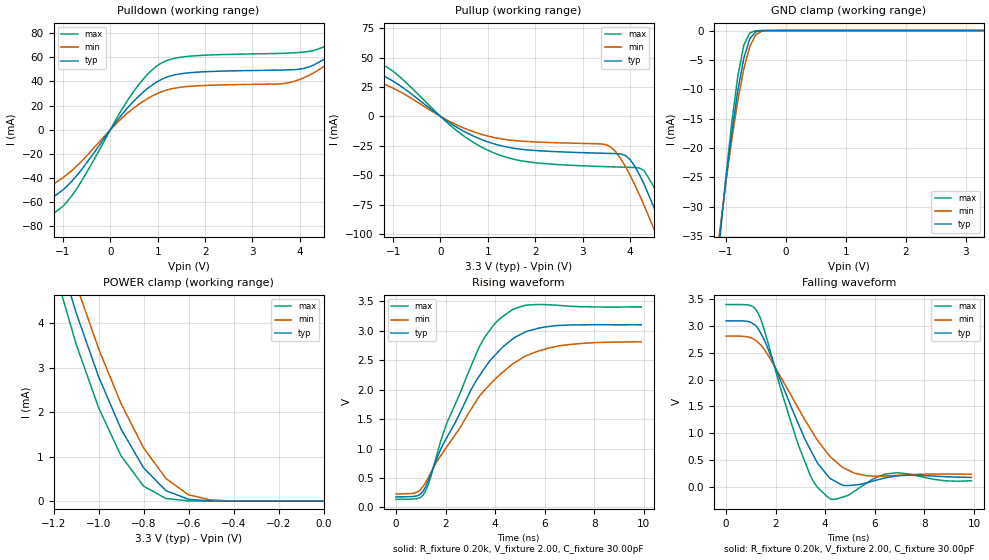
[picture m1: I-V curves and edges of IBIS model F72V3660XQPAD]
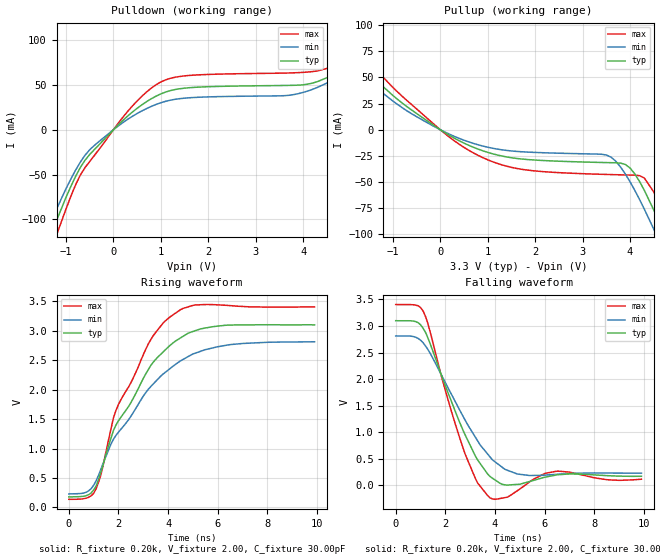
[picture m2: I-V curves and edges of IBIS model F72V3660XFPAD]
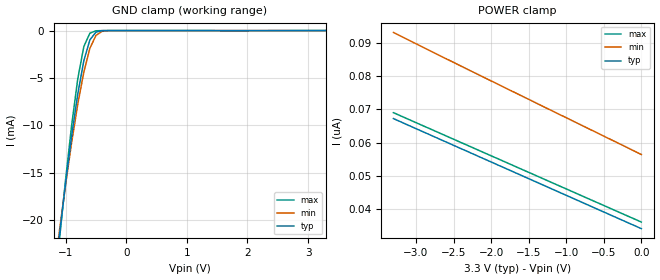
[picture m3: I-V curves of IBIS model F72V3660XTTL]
| IBIS file 72v3660p.ibs created by s2ibis2 version 1.1
| North Carolina State University Electronics Research Laboratory  1995
[IBIS ver]   2.1
[File name]   72v3660p.ibs
[File Rev]   1.0
[Date]   08/30/2001
[Source]   Integrated Device Technology, Inc.
[Notes]   1. Temperatures: typ=25C, min=85C, max=-40C 2. Cemos11.5_3v
   process. 3. Ramp rates based on 50 ohm load.
[Copyright]   Copyright 1999, Integrated Device Technology, Inc.
|   Component idt72v3660x
[Component]   idt72v3660x
[Manufacturer]   Integrated Device Technology
[Package]
| variable   typ   min   max
R_pkg   0.75   0.60   0.90
L_pkg   8.10nH   8.30nH   9.90nH
C_pkg   0.53pF   0.46pF   0.60pF
[Pin]  signal_name   model_name   R_pin   L_pin   C_pin
1   D0   F72V3660XTTL
2   D1   F72V3660XTTL
3   D2   F72V3660XTTL
4   D3   F72V3660XTTL
5   D4   F72V3660XTTL
6   D5   F72V3660XTTL
7   D6   F72V3660XTTL
8   D7   F72V3660XTTL
9   D8   F72V3660XTTL
10   D9   F72V3660XTTL
11   D10   F72V3660XTTL
12   D11   F72V3660XTTL
13   D12   F72V3660XTTL
14   D13   F72V3660XTTL
15   D14   F72V3660XTTL
16   D15   F72V3660XTTL
17   D16   F72V3660XTTL
18   D17   F72V3660XTTL
19   D18   F72V3660XTTL
20   D19   F72V3660XTTL
21   D20   F72V3660XTTL
22   D21   F72V3660XTTL
23   D22   F72V3660XTTL
24   D23   F72V3660XTTL
25   D24   F72V3660XTTL
26   D25   F72V3660XTTL
27   D26   F72V3660XTTL
28   D27   F72V3660XTTL
29   D28   F72V3660XTTL
30   D29   F72V3660XTTL
31   D30   F72V3660XTTL
32   D31   F72V3660XTTL
33   D32   F72V3660XTTL
34   D33   F72V3660XTTL
35   D34   F72V3660XTTL
36   D35   F72V3660XTTL
37   GND   GND
38   WENL   F72V3660XTTL
39   WCLK   F72V3660XTTL
40   PRSL   F72V3660XTTL
41   MRSL   F72V3660XTTL
42   LDL   F72V3660XTTL
43   FWFTSI   F72V3660XTTL
44   FFL   F72V3660XFPAD
45   PAFL   F72V3660XFPAD
46   OW   F72V3660XTTL
47   FSEL0   F72V3660XTTL
48   HFL   F72V3660XFPAD
49   FSEL1   F72V3660XTTL
50   BEL   F72V3660XTTL
51   IP   F72V3660XTTL
52   BM   F72V3660XTTL
53   ASYRL   F72V3660XTTL
54   VCC   POWER
55   PAEL   F72V3660XFPAD
56   PFM   F72V3660XTTL
57   EFL   F72V3660XFPAD
58   MARK   F72V3660XTTL
59   RCLK   F72V3660XTTL
60   RENL   F72V3660XTTL
61   RTL   F72V3660XTTL
62   OEL   F72V3660XTTL
63   Q0   F72V3660XQPAD
64   Q1   F72V3660XQPAD
65   Q2   F72V3660XQPAD
66   Q3   F72V3660XQPAD
67   Q4   F72V3660XQPAD
68   Q5   F72V3660XQPAD
69   Q6   F72V3660XQPAD
70   Q7   F72V3660XQPAD
71   Q8   F72V3660XQPAD
72   Q9   F72V3660XQPAD
73   Q10   F72V3660XQPAD
74   Q11   F72V3660XQPAD
75   Q12   F72V3660XQPAD
76   Q13   F72V3660XQPAD
77   Q14   F72V3660XQPAD
78   Q15   F72V3660XQPAD
79   Q16   F72V3660XQPAD
80   Q17   F72V3660XQPAD
81   Q18   F72V3660XQPAD
82   Q19   F72V3660XQPAD
83   Q20   F72V3660XQPAD
84   Q21   F72V3660XQPAD
85   Q22   F72V3660XQPAD
86   Q23   F72V3660XQPAD
87   Q24   F72V3660XQPAD
88   Q25   F72V3660XQPAD
89   Q26   F72V3660XQPAD
90   Q27   F72V3660XQPAD
91   Q28   F72V3660XQPAD
92   Q29   F72V3660XQPAD
93   Q30   F72V3660XQPAD
94   Q31   F72V3660XQPAD
95   Q32   F72V3660XQPAD
96   Q33   F72V3660XQPAD
97   Q34   F72V3660XQPAD
98   Q35   F72V3660XQPAD
99   TDO   F72V3660XQPAD
100   IW   F72V3660XTTL
101   SENL   F72V3660XTTL
102   ASYWL   F72V3660XTTL
| Models and submodels in the file (3): F72V3660XQPAD (3-state), F72V3660XFPAD (Output), F72V3660XTTL (Input)
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| FIN  FIN   dummy_model
| QIN  QIN   dummy_model
| QOEL QOEL   dummy_model
|   Model F72V3660XQPAD
[Model]   F72V3660XQPAD
Model_type   3-state
Polarity   Non-Inverting
Enable   Active-Low
Vinl =  0.000V
Vinh =  3.000V
Vmeas =  1.500V
C_comp   3.00pF   NA   NA
[Temperature Range]   25.00   85.00   -40.00
[Voltage Range]   3.30V   3.00V   3.60V
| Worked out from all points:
|   slope of the pulldown table from 0 to 0.495 V, typ, clamps not added: 20.9 ohm
|   slope of the pullup table from 0 to 0.495 V, typ, clamps not added: 39 ohm
|   GND clamp passes 1 mA (typ) near -0.57 V on its own axis
|   POWER clamp passes 1 mA (typ) near -0.83 V on its own axis
|   rising waveform, R_fixture 0.20k, V_fixture 2.00, C_fixture 30.00pF: 20-80 % time 2.26ns typ, 2.7ns min, 1.81ns max; typ from 0.179 V to 3.1 V
|   falling waveform, R_fixture 0.20k, V_fixture 2.00, C_fixture 30.00pF: 20-80 % time 1.58ns typ, 1.99ns min, 1.27ns max; typ from 3.1 V to 0.172 V
[Pulldown]
| voltage   I(typ)   I(min)   I(max)
-3.3V     -78.1mA    -69.1mA    -88.4mA
-1.9V     -70.5mA    -59.2mA    -83.7mA
-1.5V     -64.03mA   -52.53mA   -78.38mA
-1V       -49.8mA    -39.74mA   -63.32mA
-600mV    -32.63mA   -25.8mA    -41.94mA
400mV     19.75mA    15.01mA    26.5mA
1.1V      42.09mA    31.72mA    55.68mA
3.8V      49.61mA    39.21mA    63.53mA
4.5V      58.01mA    52.1mA     68.44mA
4.9V      71.41mA    65.07mA    81.85mA
5.3V      92.34mA    83.36mA    107mA
6.6V      239mA      203mA      293mA
[Pullup]
| voltage   I(typ)   I(min)   I(max)
-3.3V     63.83mA    53.96mA    75.83mA
-1.5V     40.98mA    32.98mA    51.93mA
300mV     -8.18mA    -6.429mA   -10.76mA
1.1V      -22.96mA   -17.67mA   -30.55mA
1.9V      -28.69mA   -21.5mA    -38.93mA
3.5V      -31.4mA    -24.13mA   -42.74mA
4V        -36.59mA   -49.74mA   -43.32mA
4.3V      -57.78mA   -75.78mA   -46.12mA
4.5V      -76.76mA   -95.06mA   -59.46mA
4.7V      -97.6mA    -115mA     -79.6mA
4.9V      -119mA     -136mA     -102mA
6.6V      -313mA     -320mA     -309mA
[GND_clamp]
| voltage   I(typ)   I(min)   I(max)
-3.3V     -278mA     -262mA     -298mA
-1.1V     -34.79mA   -34.08mA   -35.63mA
-1V       -25.68mA   -25.97mA   -25.14mA
-900mV    -17.4mA    -18.54mA   -15.66mA
-800mV    -10.26mA   -11.98mA   -7.802mA
-700mV    -4.731mA   -6.568mA   -2.51mA
-600mV    -1.413mA   -2.718mA   -390uA
-500mV    -228uA     -719uA     -31.26uA
-400mV    -22.15uA   -115uA     -1.32uA
-300mV    -1.402uA   -12.89uA   -32.97nA
3.3V      34.83nA    488nA      33.01nA
[POWER_clamp]
| voltage   I(typ)   I(min)   I(max)
-3.3V     72.27mA    66.54mA    80.97mA
-1.2V     5.92mA     6.51mA     5.285mA
-1.1V     4.244mA    4.879mA    3.539mA
-1V       2.802mA    3.433mA    2.105mA
-900mV    1.623mA    2.194mA    1.02mA
-800mV    751uA      1.201mA    338uA
-700mV    234uA      506uA      58.4uA
-600mV    41.73uA    142uA      5.351uA
-500mV    4.842uA    25.8uA     348nA
-400mV    454nA      3.649uA    51.06nA
0V        34.83nA    78.19nA    36.01nA
[Ramp]
| variable   typ   min   max
dV/dt_r   0.86/0.74n   0.65/0.97n   1.13/0.58n
dV/dt_f   1.29/0.94n   1.02/1.24n   1.58/0.64n
R_load = 50.00
[Rising Waveform]
R_fixture = 0.20k
V_fixture = 2.00
C_fixture = 30.00pF
R_dut = 0.75
L_dut = 8.10nH
C_dut = 0.53pF
| time   V(typ)   V(min)   V(max)
0s        179mV      229mV      137mV
800ps     191mV      250mV      146mV
1.1ns     281mV      361mV      211mV
1.3ns     446mV      500mV      381mV
2ns       1.146V     996mV      1.368V
3.3ns     2.193V     1.848V     2.668V
4.2ns     2.677V     2.256V     3.205V
5.2ns     2.973V     2.564V     3.43V
6.2ns     3.073V     2.71V      3.439V
9.9ns     3.1V       2.812V     3.404V
[Falling Waveform]
R_fixture = 0.20k
V_fixture = 2.00
C_fixture = 30.00pF
R_dut = 0.75
L_dut = 8.10nH
C_dut = 0.53pF
| time   V(typ)   V(min)   V(max)
0s        3.1V       2.813V     3.405V
1ns       3.071V     2.783V     3.384V
1.3ns     2.949V     2.691V     3.236V
1.8ns     2.45V      2.375V     2.505V
3ns       1.083V     1.394V     676mV
3.5ns     603mV      1.006V     116mV
4.2ns     150mV      560mV      -231mV
5.2ns     30.62mV    247mV      -80.64mV
6.5ns     169mV      199mV      239mV
9.9ns     172mV      230mV      109mV
|   Model F72V3660XFPAD
[Model]   F72V3660XFPAD
Model_type   Output
Polarity   Non-Inverting
Enable   Active-Low
Vinl =  0.000V
Vinh =  3.000V
Vmeas =  1.500V
C_comp   3.00pF   NA   NA
[Temperature Range]   25.00   85.00   -40.00
[Voltage Range]   3.30V   3.00V   3.60V
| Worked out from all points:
|   slope of the pulldown table from 0 to 0.495 V, typ, clamps not added: 20.9 ohm
|   slope of the pullup table from 0 to 0.495 V, typ, clamps not added: 39 ohm
|   rising waveform, R_fixture 0.20k, V_fixture 2.00, C_fixture 30.00pF: 20-80 % time 2.1ns typ, 2.51ns min, 1.75ns max; typ from 0.179 V to 3.1 V
|   falling waveform, R_fixture 0.20k, V_fixture 2.00, C_fixture 30.00pF: 20-80 % time 1.49ns typ, 1.82ns min, 1.2ns max; typ from 3.1 V to 0.172 V
[Pulldown]
| voltage   I(typ)   I(min)   I(max)
-3.3V     -2.813A    -331mA     -386mA
-1.5V     -140mA     -123mA     -161mA
-1V       -75.48mA   -65.71mA   -88.46mA
-700mV    -42.28mA   -36.27mA   -50.74mA
-500mV    -27.61mA   -22.34mA   -35.37mA
400mV     19.75mA    15.01mA    26.5mA
1.1V      42.09mA    31.72mA    55.68mA
4V        50.16mA    41.67mA    64.04mA
4.9V      71.41mA    65.07mA    81.85mA
5.3V      92.34mA    83.36mA    107mA
5.7V      123mA      109mA      145mA
6.6V      239mA      203mA      293mA
[Pullup]
| voltage   I(typ)   I(min)   I(max)
-3.3V     136mA      120mA      157mA
-2.5V     97.91mA    85.33mA    115mA
-2.1V     79.57mA    68.81mA    94.27mA
-700mV    21.96mA    17.97mA    27.81mA
900mV     -20.19mA   -15.64mA   -26.76mA
3.5V      -31.4mA    -24.13mA   -42.74mA
4V        -36.59mA   -49.74mA   -43.32mA
4.3V      -57.78mA   -75.78mA   -46.12mA
4.5V      -76.76mA   -95.06mA   -59.46mA
4.7V      -97.6mA    -115mA     -79.6mA
4.9V      -119mA     -136mA     -102mA
6.6V      -313mA     -320mA     -309mA
[Ramp]
| variable   typ   min   max
dV/dt_r   0.86/0.44n   0.65/0.52n   1.13/0.39n
dV/dt_f   1.29/0.69n   1.02/0.88n   1.58/0.51n
R_load = 50.00
[Rising Waveform]
R_fixture = 0.20k
V_fixture = 2.00
C_fixture = 30.00pF
R_dut = 0.75
L_dut = 8.10nH
C_dut = 0.53pF
| time   V(typ)   V(min)   V(max)
0s        179mV      229mV      137mV
1ns       297mV      375mV      239mV
1.3ns     609mV      657mV      565mV
1.8ns     1.31V      1.159V     1.524V
2ns       1.471V     1.278V     1.749V
3.3ns     2.41V      2.052V     2.849V
4.1ns     2.76V      2.365V     3.242V
5ns       2.988V     2.606V     3.431V
6ns       3.079V     2.729V     3.44V
9.9ns     3.1V       2.813V     3.404V
[Falling Waveform]
R_fixture = 0.20k
V_fixture = 2.00
C_fixture = 30.00pF
R_dut = 0.75
L_dut = 8.10nH
C_dut = 0.53pF
| time   V(typ)   V(min)   V(max)
0s        3.1V       2.813V     3.405V
800ps     3.084V     2.79V      3.394V
1.1ns     2.961V     2.688V     3.286V
2.8ns     948mV      1.226V     586mV
3.3ns     480mV      839mV      46.94mV
3.8ns     167mV      536mV      -235mV
4.3ns     19.09mV    338mV      -238mV
4.9ns     19.4mV     215mV      -100mV
6.5ns     199mV      209mV      268mV
9.9ns     172mV      230mV      117mV
|   Model F72V3660XTTL
[Model]   F72V3660XTTL
Model_type   Input
Vinl =  0.000V
Vinh =  3.000V
Vmeas =  1.500V
C_comp   3.00pF   NA   NA
[Temperature Range]   25.00   85.00   -40.00
[Voltage Range]   3.30V   3.00V   3.60V
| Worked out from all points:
|   GND clamp passes 1 mA (typ) near -0.60 V on its own axis
[GND_clamp]
| voltage   I(typ)   I(min)   I(max)
-3.3V     -163mA     -152mA     -175mA
-1.2V     -27.14mA   -26.04mA   -28.44mA
-1.1V     -21.44mA   -20.99mA   -21.88mA
-1V       -16.05mA   -16.21mA   -15.65mA
-900mV    -11.07mA   -11.76mA   -9.94mA
-800mV    -6.681mA   -7.76mA    -5.083mA
-700mV    -3.176mA   -4.372mA   -1.687mA
-600mV    -978uA     -1.868mA   -273uA
-500mV    -164uA     -509uA     -22.75uA
-400mV    -16.27uA   -84.16uA   -951nA
-300mV    -1.023uA   -9.558uA   -24.55nA
3.3V      34.02nA    59.73nA    33.01nA
[POWER_clamp]
| voltage   I(typ)   I(min)   I(max)
-3.3V     67.23nA    93.23nA    69.01nA
-2.9V     63.2nA     88.67nA    65.01nA
-2.3V     57.16nA    81.94nA    59.01nA
0V        34.02nA    56.39nA    36.01nA
